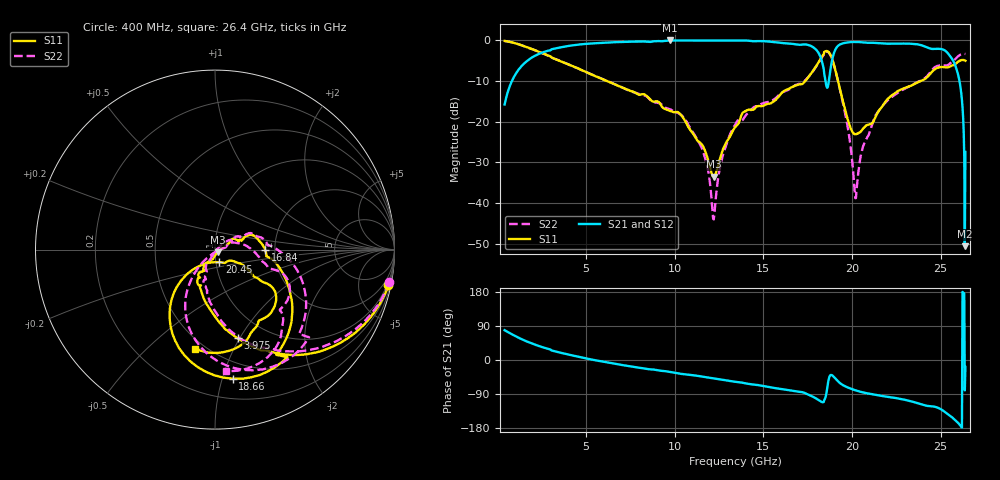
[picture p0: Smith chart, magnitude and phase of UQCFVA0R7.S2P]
!  Part Number  UQCFVA0R7  Mounting Orientation: Horizontal
!  Description: Ultra Low ESR Microwave capacitors
!  Application: Coupling, Bypass, Tuning, DC Block
!  Filters, Matching
# GHZ S DB R 50
! Freq  |S11|  S11 Ph  |S21|  S21 Ph  |S12|  S12 Ph  |S22|  S22 Ph
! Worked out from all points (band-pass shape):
!   801 points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, 400 MHz to 26.4 GHz, reference 50 ohm
!   highest |S21| = 0.00 dB at 9.728 GHz (marker M1); lowest = -50.6 dB at 26.37 GHz (marker M2)
!   |S21| within 3 dB of the highest: 2.518 GHz to 18.1 GHz (15.59 GHz wide, 151 % of centre); 18.99 GHz to 25.38 GHz (6.389 GHz wide, 28.8 % of centre)
!   lowest |S11| = -33.5 dB at 12.2 GHz (marker M3), VSWR 1.04, Z = 51.5 - j1.56 ohm
!   |S11| at or under -10 dB: 6.192 GHz to 17.36 GHz (11.17 GHz wide, 94.9 % of centre); 19.22 GHz to 23.89 GHz (4.672 GHz wide, 21.7 % of centre)
!   |S22| runs from -44.1 to -0.1 dB; largest |S21 - S12| = 0.0027
!   S11 on the Smith chart (normalised r, x): 400 MHz: 0.67, -9.79; 3.975 GHz: 0.73, -0.98; 16.84 GHz: 1.77, -0.01; 18.66 GHz: 0.36, -1.08; 20.45 GHz: 1.04, -0.15; 26.4 GHz: 0.44, -0.72
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0.4  -0.12 -11.6  -15.76 78.7  -15.76 78.7  -0.13 -10.6
1.57  -1.50 -40.6  -5.39 50.6  -5.39 50.6  -1.51 -37.9
3.975  -5.85 -75.8  -1.36 14.7  -1.35 14.8  -5.83 -74.6
4.755  -7.31 -84.0  -0.94 6.6  -0.93 6.6  -7.32 -81.9
9.078  -15.10 -121.3  -0.15 -27.6  -0.15 -27.6  -15.41 -107.7
9.728  -17.35 -118.4  0.00 -31.5  0.00 -31.5  -16.93 -109.5
11.483  -25.34 -101.5  -0.01 -43.4  -0.01 -43.4  -26.06 -114.6
12.198  -33.55 -46.2  -0.01 -48.9  -0.01 -48.8  -44.07 -36.4
12.685  -27.20 8.8  -0.01 -52.1  -0.01 -52.1  -28.81 33.5
13.4  -21.42 24.4  -0.01 -57.4  -0.01 -57.4  -20.86 34.4
16.845  -11.08 -0.6  -0.95 -82.7  -0.96 -82.7  -10.93 10.2
17.755  -7.77 -20.3  -1.52 -96.0  -1.52 -95.9  -7.85 -6.2
18.275  -4.20 -48.2  -4.69 -110.2  -4.69 -110.3  -4.34 -33.4
18.665  -2.78 -82.2  -10.86 -55.9  -10.85 -55.8  -2.87 -68.3
19.12  -8.28 -129.7  -1.81 -52.0  -1.81 -52.0  -8.35 -115.6
20.16  -23.09 -93.9  -0.36 -79.5  -0.37 -79.4  -37.61 -86.4
20.453  -22.57 -71.0  -0.41 -83.5  -0.40 -83.5  -29.47 4.5
22.078  -14.15 -30.2  -0.79 -97.4  -0.79 -97.4  -14.51 3.7
25.588  -6.28 -61.4  -4.16 -149.1  -4.16 -149.1  -5.44 -44.9
26.108  -4.94 -80.4  -11.04 -172.5  -10.99 -172.2  -3.52 -63.9
26.368  -4.93 -98.9  -50.65 -80.1  -51.43 -60.8  -3.31 -82.2
26.4  -5.00 -101.5  -27.45 -18.3  -27.41 -18.1  -3.34 -84.7
